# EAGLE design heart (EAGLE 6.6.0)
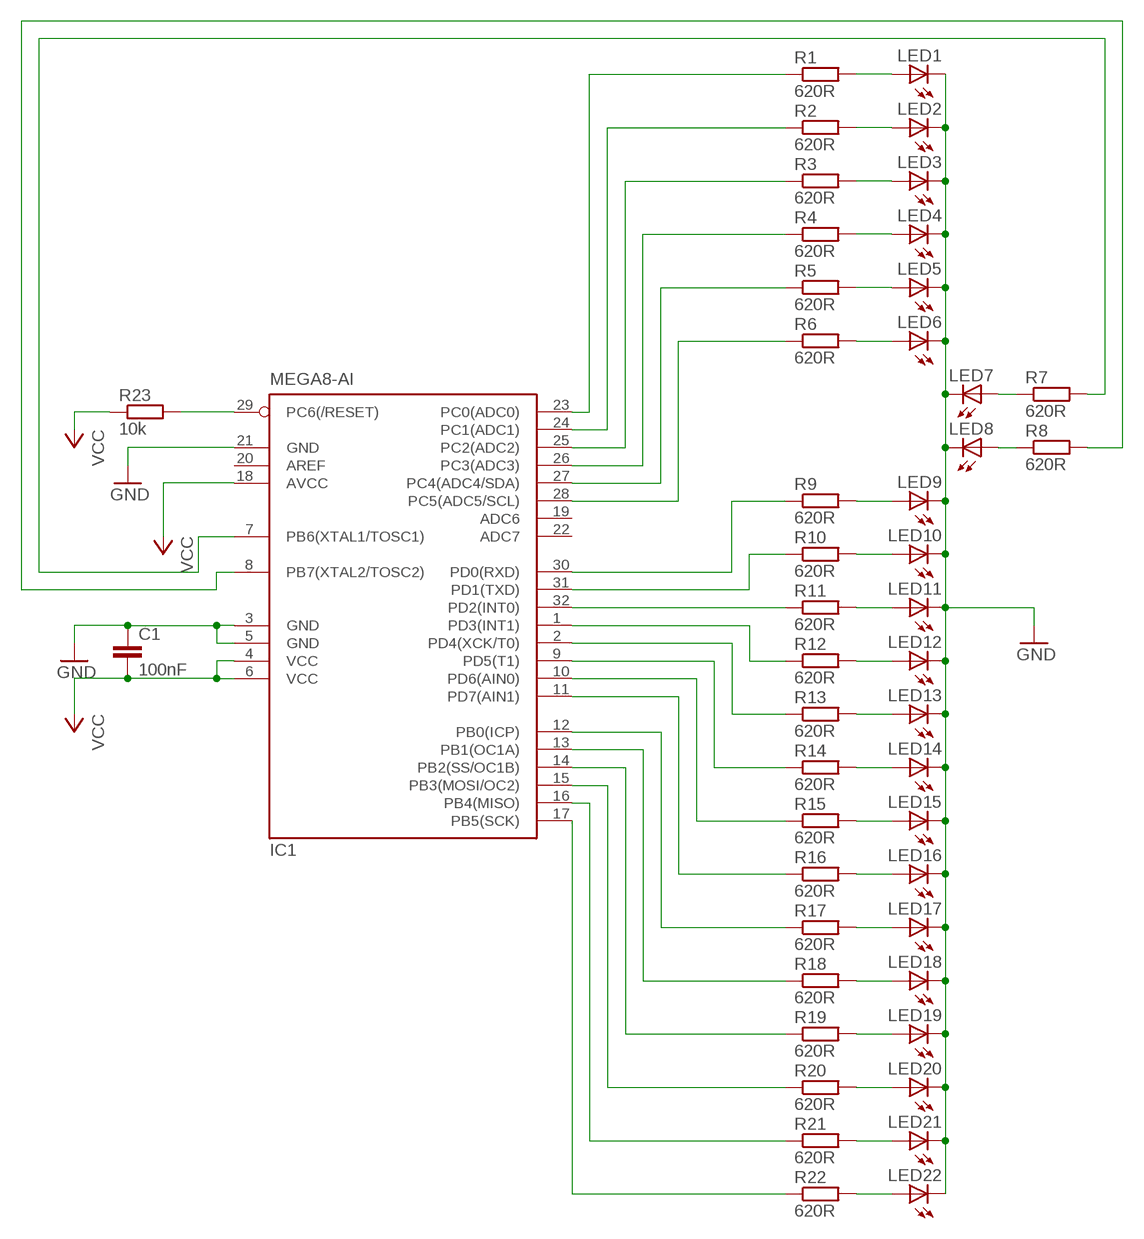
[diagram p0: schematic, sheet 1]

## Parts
C1  100nF  C-EUC0805  [C0805]
IC1  MEGA8-AI  [TQFP32-08]
LED1  LEDSML0805  [SML0805]
LED2  LEDSML0805  [SML0805]
LED3  LEDSML0805  [SML0805]
LED4  LEDSML0805  [SML0805]
LED5  LEDSML0805  [SML0805]
LED6  LEDSML0805  [SML0805]
LED7  LEDSML0805  [SML0805]
LED8  LEDSML0805  [SML0805]
LED9  LEDSML0805  [SML0805]
LED10  LEDSML0805  [SML0805]
LED11  LEDSML0805  [SML0805]
LED12  LEDSML0805  [SML0805]
LED13  LEDSML0805  [SML0805]
LED14  LEDSML0805  [SML0805]
LED15  LEDSML0805  [SML0805]
LED16  LEDSML0805  [SML0805]
LED17  LEDSML0805  [SML0805]
LED18  LEDSML0805  [SML0805]
LED19  LEDSML0805  [SML0805]
LED20  LEDSML0805  [SML0805]
LED21  LEDSML0805  [SML0805]
LED22  LEDSML0805  [SML0805]
R1  620R  R-EU_M0805  [M0805]
R2  620R  R-EU_M0805  [M0805]
R3  620R  R-EU_M0805  [M0805]
R4  620R  R-EU_M0805  [M0805]
R5  620R  R-EU_M0805  [M0805]
R6  620R  R-EU_M0805  [M0805]
R7  620R  R-EU_M0805  [M0805]
R8  620R  R-EU_M0805  [M0805]
R9  620R  R-EU_M0805  [M0805]
R10  620R  R-EU_M0805  [M0805]
R11  620R  R-EU_M0805  [M0805]
R12  620R  R-EU_M0805  [M0805]
R13  620R  R-EU_M0805  [M0805]
R14  620R  R-EU_M0805  [M0805]
R15  620R  R-EU_M0805  [M0805]
R16  620R  R-EU_M0805  [M0805]
R17  620R  R-EU_M0805  [M0805]
R18  620R  R-EU_M0805  [M0805]
R19  620R  R-EU_M0805  [M0805]
R20  620R  R-EU_M0805  [M0805]
R21  620R  R-EU_M0805  [M0805]
R22  620R  R-EU_M0805  [M0805]
R23  10k  R-EU_M0805  [M0805]

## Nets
GND: C1.1 IC1.3(GND) IC1.5(GND) IC1.21(GND) LED1.C LED2.C LED3.C LED4.C LED5.C LED6.C LED7.C LED8.C LED9.C LED10.C LED11.C LED12.C LED13.C LED14.C LED15.C LED16.C LED17.C LED18.C LED19.C LED20.C LED21.C LED22.C
N$1: LED1.A R1.2
N$2: LED2.A R2.2
N$3: LED3.A R3.2
N$4: LED4.A R4.2
N$5: LED5.A R5.2
N$6: IC1.11(PD7(AIN1)) R16.1
N$7: IC1.23(PC0(ADC0)) R1.1
N$8: IC1.29(PC6(/RESET)) R23.2
N$9: IC1.24(PC1(ADC1)) R2.1
N$10: IC1.25(PC2(ADC2)) R3.1
N$11: IC1.26(PC3(ADC3)) R4.1
N$12: IC1.27(PC4(ADC4/SDA)) R5.1
N$13: IC1.28(PC5(ADC5/SCL)) R6.1
N$14: LED7.A R7.1
N$15: LED8.A R8.1
N$16: IC1.30(PD0(RXD)) R9.1
N$17: IC1.31(PD1(TXD)) R10.1
N$18: IC1.32(PD2(INT0)) R11.1
N$19: IC1.7(PB6(XTAL1/TOSC1)) R7.2
N$20: IC1.1(PD3(INT1)) R12.1
N$21: IC1.2(PD4(XCK/T0)) R13.1
N$22: IC1.9(PD5(T1)) R14.1
N$23: IC1.10(PD6(AIN0)) R15.1
N$24: IC1.12(PB0(ICP)) R17.1
N$25: IC1.13(PB1(OC1A)) R18.1
N$26: IC1.14(PB2(SS/OC1B)) R19.1
N$27: IC1.15(PB3(MOSI/OC2)) R20.1
N$28: IC1.16(PB4(MISO)) R21.1
N$29: IC1.17(PB5(SCK)) R22.1
N$30: LED6.A R6.2
N$31: IC1.8(PB7(XTAL2/TOSC2)) R8.2
N$33: LED9.A R9.2
N$34: LED10.A R10.2
N$35: LED11.A R11.2
N$36: LED12.A R12.2
N$37: LED13.A R13.2
N$38: LED14.A R14.2
N$39: LED15.A R15.2
N$40: LED16.A R16.2
N$41: LED17.A R17.2
N$42: LED18.A R18.2
N$43: LED19.A R19.2
N$44: LED20.A R20.2
N$45: LED21.A R21.2
N$46: LED22.A R22.2
VCC: C1.2 IC1.4(VCC) IC1.6(VCC) IC1.18(AVCC) R23.1
Unconnected: IC1.19(ADC6) IC1.20(AREF) IC1.22(ADC7)

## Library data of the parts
C1 = rcl:C-EU: CAPACITOR, European symbol
IC1 = atmel:MEGA8: MICROCONTROLLER 8 Kbytes FLASH, 1 kbytes SRAM, 512 bytes EEPROM, USART, 6-channel 10 bit ADC, 2-channel 8 bit ADC Pin compatible with Atmega48, ATMega88, ATMega168 Source: avr.lbr; MPN: ATMEGA8-16AU; OC_FARNELL: 9171371; OC_NEWARK: 73M8863
LED1-LED22 = led:LED: LED
R1-R23 = resistor:R-EU_: RESISTOR, European symbol

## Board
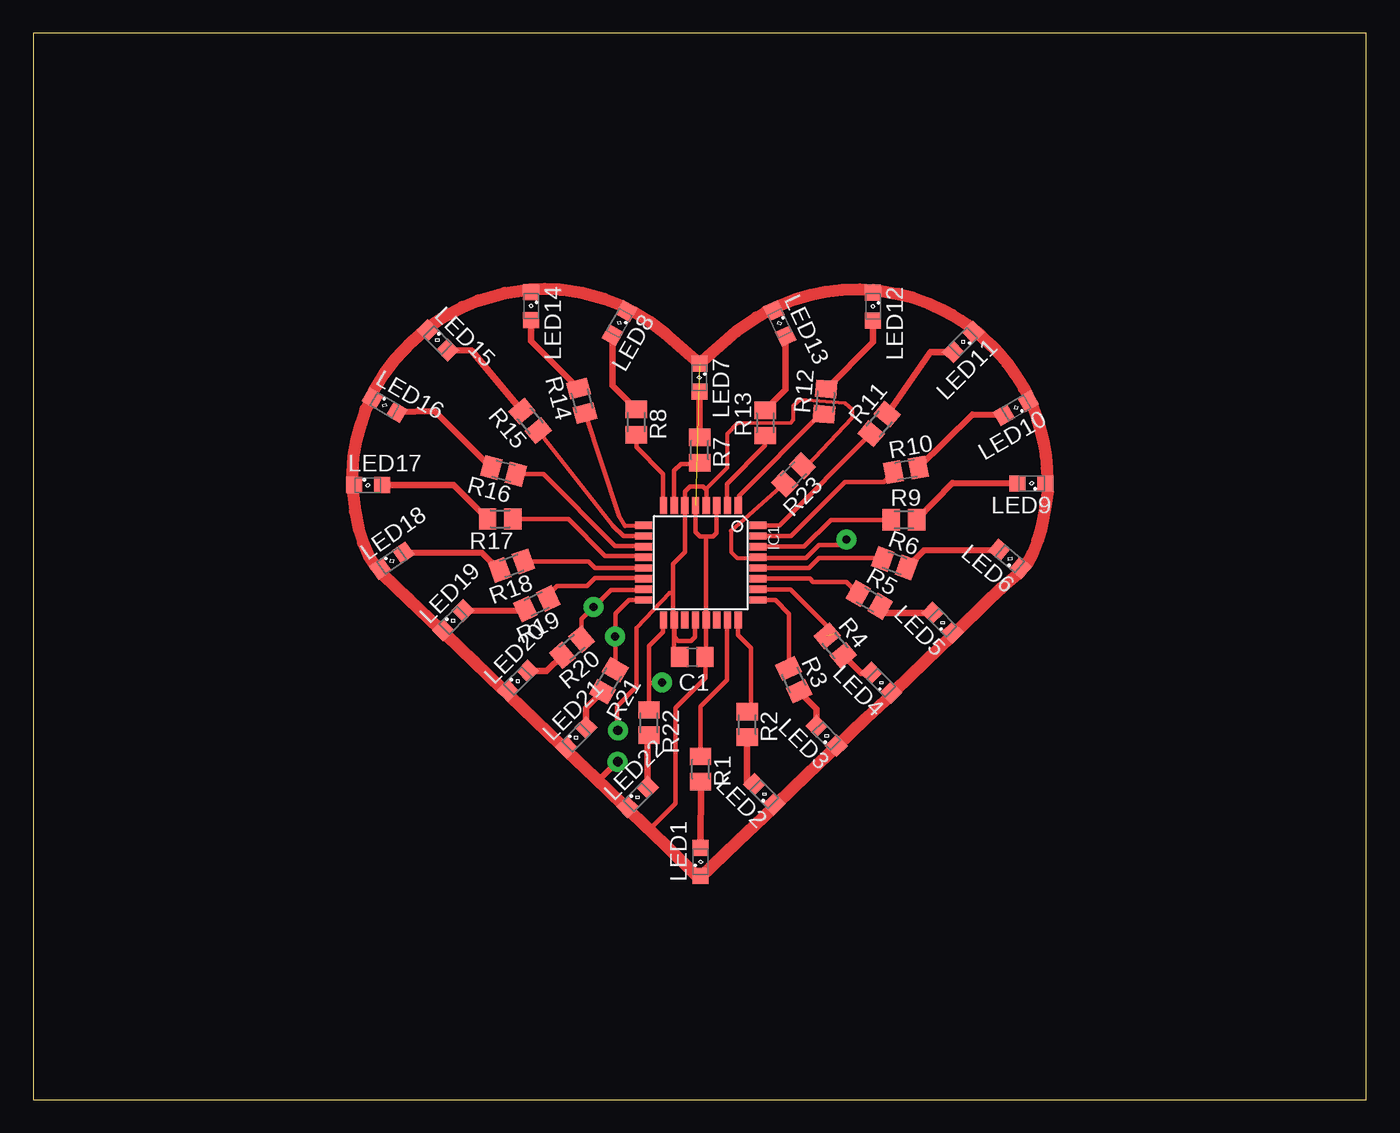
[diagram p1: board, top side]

Size 100 x 80 mm. Coordinates in mm from the lower left corner, seen from the top.
Outline: 100,0 100,80 0,80 0,0 100,0
Copper layers (1*16): Top 0.035mm / dielectric 1.5mm / Bottom 0.035mm
Design rules "default": minimum track width 20mil, minimum drill 32mil, track to track 12mil, track to pad 12mil, pad to pad 12mil, via to via 12mil, smd to smd 8mil, copper to edge 40mil, drill to drill 40mil, minimum pad ring 25mil, minimum via ring 12mil, stop-mask expansion 4mil, vias tented up to drill 0mil, thermal gap 10mil

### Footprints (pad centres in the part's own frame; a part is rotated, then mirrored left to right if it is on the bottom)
C0805 = smd 1.3 x 1.5: 1 -0.95,0; 2 0.95,0
TQFP32-08 = smd 1.27 x 0.559: 1 -4.293,2.8; 2 -4.293,2; 3 -4.293,1.2; 4 -4.293,0.4; 5 -4.293,-0.4; 6 -4.293,-1.2; 7 -4.293,-2; 8 -4.293,-2.8; 17 4.293,-2.8; 18 4.293,-2; 19 4.293,-1.2; 20 4.293,-0.4; 21 4.293,0.4; 22 4.293,1.2; 23 4.293,2; 24 4.293,2.8 | smd 0.559 x 1.27: 9 -2.8,-4.293; 10 -2,-4.293; 11 -1.2,-4.293; 12 -0.4,-4.293; 13 0.4,-4.293; 14 1.2,-4.293; 15 2,-4.293; 16 2.8,-4.293; 25 2.8,4.293; 26 2,4.293; 27 1.2,4.293; 28 0.4,4.293; 29 -0.4,4.293; 30 -1.2,4.293; 31 -2,4.293; 32 -2.8,4.293
SML0805 = smd 1.2 x 1.2: A 1.05,0; C -1.05,0
M0805 = smd 1.3 x 1.6: 1 -0.95,0; 2 0.95,0

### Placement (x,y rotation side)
C1  49.44,33.19 180 top
IC1  50.08,40.28 270 top
LED1  50.05,17.85 90 top
LED2  54.84,22.91 135 top
LED3  59.51,27.28 135 top
LED4  63.61,31.28 135 top
LED5  68.21,35.78 135 top
LED6  73.27,40.57 140 top
LED7  49.97,54.16 270 top
LED8  43.97,58.26 240 top
LED9  74.89,46.22 180 top
LED10  73.73,51.89 210 top
LED11  69.77,56.84 225 top
LED12  63,59.51 270 top
LED13  56,58.24 295 top
LED14  37.35,59.53 270 top
LED15  30.33,56.97 315 top
LED16  26.36,52.09 330 top
LED17  25.11,46.1 0 top
LED18  26.9,40.43 35 top
LED19  31.5,35.95 45 top
LED20  36.35,31.41 45 top
LED21  40.73,27.16 45 top
LED22  45.34,22.68 45 top
R1  50.06,24.79 270 top
R2  53.56,28.14 270 top
R3  57.06,31.49 295 top
R4  60.16,34.06 310 top
R5  62.72,37.49 330 top
R6  64.62,40.24 340 top
R7  49.99,48.73 270 top
R8  45.24,50.83 270 top
R9  65.32,43.49 0 top
R10  65.47,47.24 10 top
R11  63.46,50.69 50 top
R12  59.41,52.37 85 top
R13  54.91,50.77 90 top
R14  41.16,52.42 105 top
R15  37.27,50.91 130 top
R16  35.28,47.16 165 top
R17  35.03,43.56 180 top
R18  35.88,40.06 200 top
R19  37.77,37.19 205 top
R20  40.42,33.94 220 top
R21  43.19,31.43 240 top
R22  46.19,28.28 270 top
R23  57.04,46.88 225 top

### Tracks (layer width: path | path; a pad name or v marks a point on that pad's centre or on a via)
GND  (1 unrouted)
  Top 0.35: IC1.5 49.68,42.57 50,42.25 50.4,42.25 | 50.4,42.25 51,42.25 51.25,42.5 51.25,44.54 IC1.3 | 50.4,42.25 50.48,42.17 IC1.21 50.48,33.28 C1.1
  Top 0.9: 64.45,30.54 LED4.C | 60.35,26.54 LED3.C | LED4.C 64.61,30.61 66.84,32.8 68.92,34.79 LED5.C 69.44,35.28 71.31,37.09 72.64,38.37 74.04,39.59 LED6.C 74.14,39.85 74.56,40.2 74.95,40.95 75.33,41.92 75.62,42.91 75.93,44.55 76.1,45.74 LED9.C 76.08,46.53 76.04,47.35 75.95,48.28 75.77,49.34 75.57,50.2 75.33,50.99 74.87,52.28 LED10.C 74.61,52.77 74.3,53.38 73.64,54.45 73.07,55.24 72.61,55.81 71.93,56.55 71.06,57.37 70.64,57.7 LED11.C 70.42,57.87 70.11,58.11 69.57,58.48 68.95,58.86 68.23,59.25 67.22,59.71 65.93,60.19 64.92,60.45 63.5,60.68 LED12.C 63.03,60.74 62,60.8 60.69,60.76 59.42,60.61 58.35,60.39 57.16,60.04 55.87,59.53 LED13.C 55,59.12 54.25,58.67 52.77,57.64 LED7.C 47.36,57.52 46.28,58.35 44.98,59.11 LED8.C 44.11,59.56 42.83,60.07 41.17,60.52 39.52,60.76 38.38,60.81 37.19,60.76 LED14.C 36.85,60.73 35.36,60.52 33.38,59.96 32.19,59.46 30.89,58.77 29.93,58.13 LED15.C 29.03,57.45 28.37,56.84 27.13,55.51 26.3,54.42 25.51,53.07 LED16.C 25.09,52.04 24.93,51.77 24.58,50.69 24.24,49.5 24.03,48.25 23.92,46.42 LED17.C 23.95,45.66 24.14,44.14 24.42,42.79 24.74,41.79 25.17,40.78 25.67,40.01 LED18.C 26.22,39.44 28.17,37.57 30.53,35.3 LED19.C 30.97,34.9 33.07,32.87 35.26,30.78 LED20.C 35.73,30.33 37.65,28.48 39.68,26.54 LED21.C 40.09,26.13 42.13,24.17 44.27,22.11 LED22.C | LED4.C 64.43,30.41 62.44,28.56 60.23,26.43 LED3.C | LED3.C 60.49,26.69 57.99,24.31 55.77,22.16 LED2.C 55.48,21.86 52.84,19.34 49.98,16.6 LED1.C
N$1
  Top 0.5: R1.2 50.09,23.81 LED1.A
N$2
  Top 0.5: R2.2 53.55,23.7 53.6,23.65 LED2.A
N$3
  Top 0.5: R3.2 58.77,29.32 LED3.A
N$4
  Top 0.5: R4.2 62.08,32.02 LED4.A
N$5
  Top 0.5: R5.2 64.03,36.52 LED5.A
N$6
  Top 0.34: IC1.11 45.72,41.55 43.65,41.55 38.29,46.91 R16.1
N$7
  Top 0.34: IC1.23 52.05,35.96 52.05,31.5 50.06,29.51 R1.1
N$8
  Top 0.3: R23.2 52.34,42.66 52.35,41.1 52.8,40.65 54.34,40.65 IC1.29
N$9
  Top 0.34: IC1.24 52.88,34.87 53.85,33.9 53.85,29.38 R2.1
N$10
  Top 0.34: IC1.25 55.67,37.48 56.7,36.45 56.7,32.39 R3.1
N$11  (1 unrouted)
  Top 0.34: IC1.26 56.82,38.28 60.15,34.95
N$12
  Top 0.34: IC1.27 58.27,39.08 58.5,38.85 61.01,38.85 R5.1
N$13
  Top 0.34: IC1.28 58.18,39.88 58.95,40.65 63.64,40.65 R6.1
N$14
  Top 0.5: LED7.A 49.97,49.7 R7.1
N$15
  Top 0.5: R8.1 43.45,53.58 LED8.A
N$16
  Top 0.34: IC1.30 57.83,41.48 59.85,43.5 R9.1
N$17
  Top 0.34: IC1.31 56.83,42.28 60.9,46.35 63.81,46.35 R10.1
N$18
  Top 0.34: IC1.32 55.97,43.08 R11.1
N$19
  Top 0.34: IC1.7 48.08,47.18 48.6,47.7 49.91,47.7 R7.2
N$20
  Top 0.34: IC1.1 52.95,44.64 52.95,45.3 59.07,51.42 R12.1
N$21
  Top 0.34: R13.1 54.91,49.06 52.05,46.2 52.05,44.6 IC1.2
N$22
  Top 0.34: R14.1 43.95,43.8 44.4,43.05 IC1.9
N$23
  Top 0.34: IC1.10 44.27,42.28 43.5,43.05 R15.1
N$24
  Top 0.34: IC1.12 45.67,40.8 42.9,40.8 40.14,43.56 R17.1
N$25
  Top 0.34: IC1.13 45.77,39.9 42.15,39.9 41.66,40.38 R18.1
N$26
  Top 0.34: IC1.14 45.72,39.15 42.15,39.15 41.55,38.55 39.3,38.55 38.63,37.88 R19.1
N$27
  Top 0.34: IC1.15 45.76,38.25 43.35,38.25 41.15,36.05 R20.1
N$28
  Top 0.34: IC1.16 45.77,37.5 44.7,37.5 43.66,36.47 R21.1
N$29
  Top 0.34: IC1.17 47.25,35.96 47.25,35.1 46.19,34.04 46.19,31.26 R22.1
  Top 0.35: 46.19,31.26 46.99,31.26
N$30
  Top 0.5: R6.2 66.8,41.2 LED6.A
N$31
  Top 0.34: R8.2 45.24,48.96 47.25,46.95 47.25,44.6 IC1.8
N$33
  Top 0.5: R9.2 68.96,46.26 LED9.A
N$34
  Top 0.5: R10.2 70.45,51.41 LED10.A
N$35
  Top 0.5: R11.2 67.3,56.1 LED11.A
N$36
  Top 0.5: R12.2 63,56.82 LED12.A
N$37
  Top 0.5: R13.2 56.44,53.25 LED13.A
N$38
  Top 0.5: R14.2 37.35,56.9 LED14.A
N$39
  Top 0.5: R15.2 32.88,56.19 LED15.A
N$40
  Top 0.5: R16.2 30.12,51.65 LED16.A
N$41
  Top 0.5: R17.2 31.54,46.1 LED17.A
N$42
  Top 0.5: R18.2 33.67,41.02 LED18.A
N$43
  Top 0.5: R19.2 36.77,36.65 LED19.A
N$44
  Top 0.5: R20.2 38.52,32.15 LED20.A
N$45
  Top 0.5: R21.2 41.47,29.36 LED21.A
N$46
  Top 0.5: R22.2 46.08,27.22 LED22.A
N$47
  Top 0.35: 50.42,33.07 50.42,31.65 48.17,29.4 48.17,22.21 46.2,20.24
N$48  (via drill 0.7 pad 1.5)
  other vias: 43.84,25.34
N$49  (via drill 0.7 pad 1.5)
  other vias: 43.85,27.7
N$50
  Top 0.5: 43.79,25.34 42.47,24.02
N$51
  Top 0.3: 47.74,38 45.27,35.4
  Top 0.35: 48.01,38.01 47.74,38 | 45.27,35.4 45.27,30.98 43.8,29.51 43.8,27.83 43.95,27.68
N$52  (via drill 0.6 pad 1.5)
  other vias: 47.17,31.29
N$53  (via drill 0.6 pad 1.5)
  other vias: 43.65,34.73
N$54  (via drill 0.6 pad 1.5)
  other vias: 42.04,36.96
N$55  (via drill 0.6 pad 1.5)
  other vias: 60.99,42.02
N$56
  Top 0.35: 54.56,40.63 57.95,40.63 58.94,41.62 60.54,41.62 60.88,41.96
N$57
  Top 0.9: 44.56,21.99 44.84,21.58 47.45,19.07 49.98,16.61 49.96,16.77
N$58
  Top 0.35: 48.09,35.52 48.09,34.69 48.38,34.4 49.35,34.4 49.64,34.69 49.64,35.67 49.67,35.7
VCC
  Top 0: IC1.6 48.88,45.13 | 50.48,45.27 IC1.4
  Top 0.254: 60.9,52.25 57.55,52.53 | 56.82,50.76 52.83,50.75
  Top 0.3: R23.1 58.05,47.55 61.45,51.17 61.45,51.77 60.9,52.25 | 57.55,52.53 57,52.05 57,51 56.82,50.76 | 52.83,50.75 52.05,49.95 52.05,47.4 50.5,45.85 50.5,45.75
  Top 0.35: IC1.4 50.5,44.59 50.5,45.75 50.25,46 49.25,46 48.88,45.63 IC1.6 48.88,41.08 48,40.2 48,36.07 IC1.18 48.08,33.6 C1.2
